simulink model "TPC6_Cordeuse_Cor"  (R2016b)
settings: Solver=ode23t  StartTime=0.0  StopTime=5  RelTol=1e-3  EnableMultiTasking=on
model workspace (MAT data in the model file):
  J = 8e-05
  K1 = 0.561
  Kcan = 51
  Kcorde = 5052
  Ke = 0.024
  Kh = 0.0705882352941
  Ki = 0.2
  Kp = 10
  Kpc = 0.01
  Kpot = 0.333333333333
  Kr = 0.0188087774295
  Kress = 0.033
  L = 0.02
  R = 0.7
  f = 0.006
libraries: simulink x1

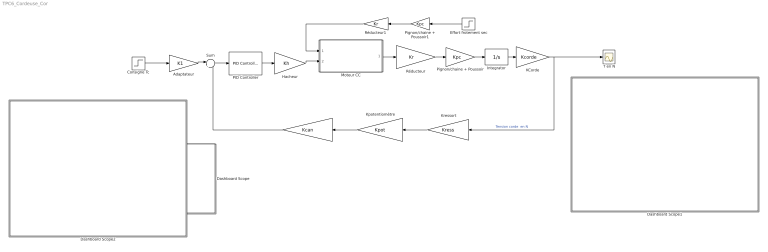
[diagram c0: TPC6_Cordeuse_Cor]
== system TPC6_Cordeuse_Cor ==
  " " : Gain  Gain=Kcan
  " Kpotentiomètre" : Gain  Gain=Kpot
  " Kressort" : Gain  Gain=Kress
  Adaptateur : Gain  Gain=K1
  Consigne Tc : Step  Time=0  After=250  SampleTime=0
  Dashboard Scope : Subsystem  DialogController=hmiCreateDDGDialog  IsWebBlock=on
  Dashboard Scope1 : Subsystem  DialogController=hmiCreateDDGDialog  IsWebBlock=on
  Dashboard Scope2 : Subsystem  DialogController=hmiCreateDDGDialog  IsWebBlock=on
  Effort frotement sec : Step  Time=0  After=127  SampleTime=0
  Hacheur : Gain  Gain=Kh
  Integrator : Integrator
  KCorde : Gain  Gain=Kcorde
  Moteur CC : Subsystem
  PID Controller : simulink/Continuous/PID Controller  Controller=PID  TimeDomain=Continuous-time  SampleTime=-1  IntegratorMethod=Forward Euler  FilterMethod=Forward Euler  Form=Parallel  UseFilter=on  ControllerParametersSource=internal  P=Kp  I=Ki  D=0  N=100  InitialConditionSource=internal  InitialConditionForIntegrator=0  InitialConditionForFilter=0  ExternalReset=none  LimitOutput=off  UpperSaturationLimit=inf  LowerSaturationLimit=-inf  LinearizeAsGain=on  AntiWindupMode=none  Kb=1  TrackingMode=off  Kt=1  PParamMin=[]  PParamMax=[]  IParamMin=[]  IParamMax=[]  DParamMin=[]  DParamMax=[]  NParamMin=[]  NParamMax=[]  KbParamMin=[]  KbParamMax=[]  KtParamMin=[]  KtParamMax=[]  POutMin=[]  POutMax=[]  IOutMin=[]  IOutMax=[]  DOutMin=[]  DOutMax=[]  NOutMin=[]  NOutMax=[]  KbOutMin=[]  KbOutMax=[]  KtOutMin=[]  KtOutMax=[]  IntegratorOutMin=[]  IntegratorOutMax=[]  FilterOutMin=[]  FilterOutMax=[]  SumOutMin=[]  SumOutMax=[]  SumI1OutMin=[]  SumI1OutMax=[]  SumI2OutMin=[]  SumI2OutMax=[]  SumI3OutMin=[]  SumI3OutMax=[]  SumDOutMin=[]  SumDOutMax=[]  SaturationOutMin=[]  SaturationOutMax=[]  IntegratorContinuousStateAttributes=''  IntegratorStateMustResolveToSignalObject=off  IntegratorRTWStateStorageClass=Auto  FilterContinuousStateAttributes=''  FilterStateMustResolveToSignalObject=off  FilterRTWStateStorageClass=Auto  DifferentiatorICPrevScaledInput=0  DifferentiatorOutMin=[]  DifferentiatorOutMax=[]
  Pignon/chaine + Poussoir : Gain  Gain=Kpc
  Pignon/chaine + Poussoir1 : Gain  Gain=Kpc
  Réducteur : Gain  Gain=Kr
  Réducteur1 : Gain  Gain=Kr
  Sum : Sum  Inputs=|+-
  T en N : Scope
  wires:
  Adaptateur/1 -> Sum/1
  Sum/1 -> PID Controller/1
  PID Controller/1 -> Hacheur/1
  Réducteur/1 -> Pignon/chaine + Poussoir/1
  Pignon/chaine + Poussoir/1 -> Integrator/1
  " "/1 -> Sum/2
  Consigne Tc/1 -> Adaptateur/1
  Integrator/1 -> KCorde/1
  " Kpotentiomètre"/1 -> " "/1
  " Kressort"/1 -> " Kpotentiomètre"/1
  Pignon/chaine + Poussoir1/1 -> Réducteur1/1
  Effort frotement sec/1 -> Pignon/chaine + Poussoir1/1
  Réducteur1/1 -> Moteur CC/1(In1)
  Hacheur/1 -> Moteur CC/2(In2)
  Moteur CC/1(Out1) -> Réducteur/1
  KCorde/1 -> T en N/1, " Kressort"/1  "Tension corde  en N"

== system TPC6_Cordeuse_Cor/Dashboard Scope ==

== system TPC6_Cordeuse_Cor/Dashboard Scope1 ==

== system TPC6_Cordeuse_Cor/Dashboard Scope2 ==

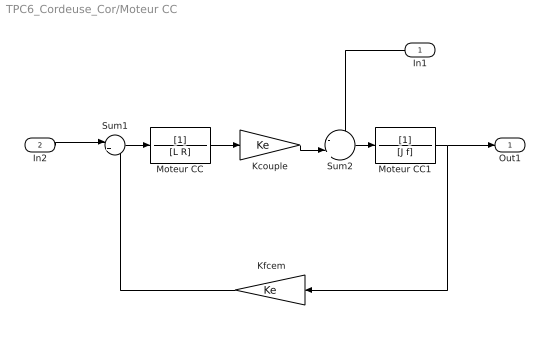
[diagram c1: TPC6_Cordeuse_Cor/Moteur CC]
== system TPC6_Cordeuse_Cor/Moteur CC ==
  In1 : Inport
  In2 : Inport  Port=2
  " Kfcem" : Gain  Gain=Ke
  Kcouple : Gain  Gain=Ke
  Moteur CC : TransferFcn  Denominator=[L R]
  Moteur CC1 : TransferFcn  Denominator=[J f]
  Sum1 : Sum  Inputs=|+-
  Sum2 : Sum  Inputs=-|+||
  Out1 : Outport
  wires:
  " Kfcem"/1 -> Sum1/2
  Moteur CC/1 -> Kcouple/1
  In2/1 -> Sum1/1
  Sum1/1 -> Moteur CC/1
  Moteur CC1/1 -> Out1/1, " Kfcem"/1
  In1/1 -> Sum2/1
  Sum2/1 -> Moteur CC1/1
  Kcouple/1 -> Sum2/2
